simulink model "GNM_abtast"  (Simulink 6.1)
settings: Solver=ode45  StartTime=0.0  StopTime=0.2  RelTol=1e-3
InitFcn:
  | GNM_abtast_ini
StopFcn:
  | GNM_abtast_plot
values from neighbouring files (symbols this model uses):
  CE = (2*NA/pi)*2*pi    (= 240)    [GNM_abtast_ini.m]
  CM = 2*NA/pi    (= 38.1971863421)    [GNM_abtast_ini.m]
  Fpwm = 5000    [GNM_abtast_ini.m]
  Imax = 20    [GNM_abtast_ini.m]
  J = 0.012    [GNM_abtast_ini.m]
  LA = 0.004    [GNM_abtast_ini.m]
  Mw = 10    [GNM_abtast_ini.m]
  N_soll = 1000 / 60    (= 16.6666666667)    [GNM_abtast_ini.m]
  psi = 0.04    [GNM_abtast_ini.m]
  RA = 0.25    [GNM_abtast_ini.m]
  TnAd = 8*Tsn/2    (= 0.0032)    [GNM_abtast_ini.m]
  Tsi = 0.0008    [GNM_abtast_ini.m]
  Tsn = 0.0008    [GNM_abtast_ini.m]
  TstrA = 1 / Fpwm / 2    (= 0.0001)    [GNM_abtast_ini.m]
  Umax = 200    [GNM_abtast_ini.m]
  VnAd = 2*pi*J/(4*Tsn/2*CM*psi)    (= 30.8425137534)    [GNM_abtast_ini.m]
undefined symbols (not defined in the file or in its folder): Ad, Bd
libraries: simulink x1

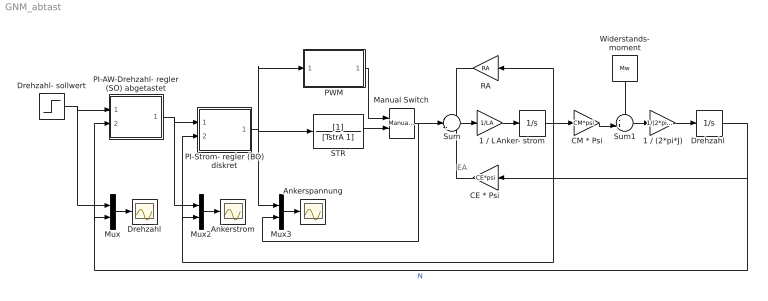
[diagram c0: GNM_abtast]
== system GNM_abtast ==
  note: EA
  " Widerstands-  moment" : Constant  Orientation=down  Value=Mw
  1 / (2*pi*J) : Gain  Gain=1/(2*pi*J)
  1 / LA : Gain  Gain=1/LA
  Anker- strom : Integrator
  Ankerspannung : Scope
  Ankerstrom : Scope
  "CE * Psi " : Gain  Orientation=left  Gain=CE*psi
  CM * Psi : Gain  Gain=CM*psi
  Drehzahl : Scope
  "Drehzahl " : Integrator
  Drehzahl- sollwert : Step  Time=0.05  After=N_soll  SampleTime=0
  Manual Switch : simulink/Signal Routing/Manual Switch  sw=0  action=0
  Mux : Mux  Inputs=2
  Mux2 : Mux  Inputs=2
  Mux3 : Mux  Inputs=2
  PI-AW-Drehzahl- regler (SO) abgetastet : Subsystem
  PI-Strom- regler (BO) diskret : Subsystem
  PWM : Subsystem
  RA : Gain  Orientation=left  Gain=RA
  STR : TransferFcn  Denominator=[TstrA 1]
  Sum : Sum  Inputs=-+-
  Sum1 : Sum  Inputs=-+|
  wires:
  RA/1 -> Sum/1
  Anker- strom/1 -> CM * Psi/1, RA/1, Mux2/2, PI-Strom- regler (BO) diskret/2(IA)
  Sum/1 -> 1 / LA/1
  1 / LA/1 -> Anker- strom/1
  CM * Psi/1 -> Sum1/2
  Sum1/1 -> 1 / (2*pi*J)/1
  1 / (2*pi*J)/1 -> "Drehzahl "/1
  " Widerstands-  moment"/1 -> Sum1/1
  "CE * Psi "/1 -> Sum/3
  PWM/1(UAist) -> Manual Switch/1
  STR/1 -> Manual Switch/2
  Mux/1 -> Drehzahl/1
  PI-AW-Drehzahl- regler (SO) abgetastet/1(IAsoll) -> PI-Strom- regler (BO) diskret/1(IAsoll), Mux2/1
  Mux2/1 -> Ankerstrom/1
  Mux3/1 -> Ankerspannung/1
  PI-Strom- regler (BO) diskret/1(UAsoll) -> Mux3/1, STR/1, PWM/1(UAsoll)
  Drehzahl- sollwert/1 -> Mux/1, PI-AW-Drehzahl- regler (SO) abgetastet/1(N_soll)
  Manual Switch/1 -> Sum/2, Mux3/2
  "Drehzahl "/1 -> "CE * Psi "/1, Mux/2, PI-AW-Drehzahl- regler (SO) abgetastet/2(N)  "N"

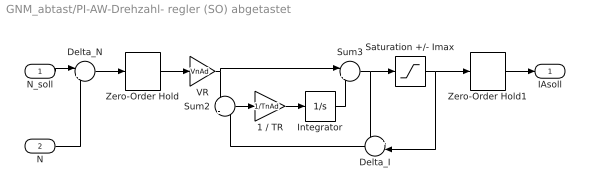
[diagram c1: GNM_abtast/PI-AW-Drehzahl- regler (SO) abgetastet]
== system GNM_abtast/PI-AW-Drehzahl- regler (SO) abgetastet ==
  N_soll : Inport  Port=1  LatchInput=off
  N : Inport  Port=2  LatchInput=off
  1 / TR : Gain  Gain=1/TnAd
  Delta_I : Sum  Orientation=left  Inputs=+-|
  Delta_N : Sum  Inputs=|+-
  Integrator : Integrator
  Saturation +/- Imax : Saturate  UpperLimit=Imax  LowerLimit=-Imax
  Sum2 : Sum  Inputs=+|-
  Sum3 : Sum  Inputs=|++
  VR : Gain  Gain=VnAd
  Zero-Order Hold : ZeroOrderHold  SampleTime=Tsn
  Zero-Order Hold1 : ZeroOrderHold  SampleTime=Tsn
  IAsoll : Outport  InitialOutput=0
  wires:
  N_soll/1 -> Delta_N/1
  N/1 -> Delta_N/2
  Delta_N/1 -> Zero-Order Hold/1
  Integrator/1 -> Sum3/2
  Sum3/1 -> Saturation +/- Imax/1, Delta_I/1
  Sum2/1 -> 1 / TR/1
  VR/1 -> Sum2/1, Sum3/1
  Delta_I/1 -> Sum2/2
  1 / TR/1 -> Integrator/1
  Saturation +/- Imax/1 -> Delta_I/2, Zero-Order Hold1/1
  Zero-Order Hold/1 -> VR/1
  Zero-Order Hold1/1 -> IAsoll/1

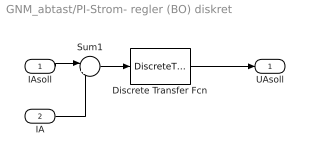
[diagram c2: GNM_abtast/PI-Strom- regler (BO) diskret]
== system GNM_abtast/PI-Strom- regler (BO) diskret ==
  IAsoll : Inport  Port=1  LatchInput=off
  IA : Inport  Port=2  LatchInput=off
  Discrete Transfer Fcn : DiscreteTransferFcn  Numerator=Bd  Denominator=Ad  SampleTime=Tsi
  Sum1 : Sum  Inputs=|+-
  UAsoll : Outport  InitialOutput=0
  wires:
  IAsoll/1 -> Sum1/1
  IA/1 -> Sum1/2
  Sum1/1 -> Discrete Transfer Fcn/1
  Discrete Transfer Fcn/1 -> UAsoll/1

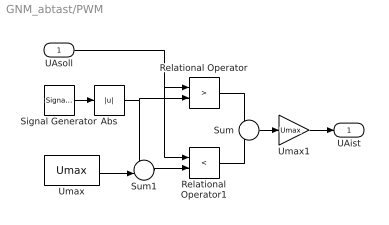
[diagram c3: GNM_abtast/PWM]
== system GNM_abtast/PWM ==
  UAsoll : Inport  Port=1  LatchInput=off
  Abs : Abs
  Relational Operator : RelationalOperator  Operator=>
  Relational Operator1 : RelationalOperator  Operator=<
  Signal Generator : SignalGenerator  WaveForm=sawtooth  Amplitude=Umax  Frequency=Fpwm
  Sum : Sum  Inputs=+-
  Sum1 : Sum  Inputs=+-|
  Umax : Constant  Value=Umax
  Umax1 : Gain  Gain=Umax
  UAist : Outport  InitialOutput=0
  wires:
  Signal Generator/1 -> Abs/1
  Sum1/1 -> Relational Operator1/2
  UAsoll/1 -> Relational Operator1/1, Relational Operator/1
  Abs/1 -> Relational Operator/2, Sum1/1
  Umax/1 -> Sum1/2
  Relational Operator/1 -> Sum/1
  Relational Operator1/1 -> Sum/2
  Umax1/1 -> UAist/1
  Sum/1 -> Umax1/1
